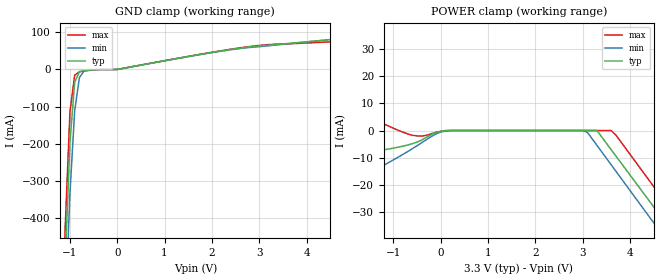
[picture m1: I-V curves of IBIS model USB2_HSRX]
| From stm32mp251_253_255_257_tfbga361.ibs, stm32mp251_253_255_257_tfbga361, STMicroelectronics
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[Model] USB2_HSRX
Model_type   Input
Polarity   Non-Inverting
Enable   Active-High
C_comp   5.492pF   5.368pF   5.494pF
Vinh = 150.000mV
Vinl = -150.000mV
[Model Spec]
[Receiver Thresholds]
Vcross_low = 0
Vcross_high = 500mv
Vdiff_ac = 150mv
Vdiff_dc = 100mv
Tdiffslew_ac = 1200ps
[Temperature Range]   25.000   125.000   -40.000
[Voltage Range]   3.300V   3.070V   3.630V
[GND Clamp Reference]   0.00V   0.00V   0.00V
[POWER Clamp Reference]   3.300V   3.070V   3.630V
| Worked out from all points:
|   GND clamp passes 1 mA (typ) near -0.53 V on its own axis
|   POWER clamp passes 1 mA (typ) near -0.14 V on its own axis
[GND Clamp]
-3.3V     -10.95A    -10.55A    -11.25A
-1.2V     -915.3mA   -1.032A    -838.8mA
-1.1V     -519.2mA   -657.5mA   -425.7mA
-1V       -197.7mA   -335.1mA   -115.1mA
-900mV    -35.05mA   -112.2mA   -15.67mA
-800mV    -5.949mA   -22.12mA   -6.454mA
-700mV    -2.647mA   -3.891mA   -4.243mA
-600mV    -1.536mA   -1.033mA   -2.639mA
1.971fV   0A         0A         0A
2V        45.55mA    45.52mA    46.3mA
3V        63.49mA    61.26mA    64.65mA
6.6V      104.1mA    107.2mA    86.72mA
[Power Clamp]
-3.3V     3.177A     2.138A     4.841A
-2.7V     505.5mA    62.8mA     1.908A
-2.6V     183.2mA    -5.843mA   1.435A
-2.4V     -6.294mA   -21.52mA   553.3mA
-2.2V     -8.53mA    -21.55mA   47.5mA
-2.1V     -8.617mA   -20.87mA   13.18mA
-2V       -8.548mA   -20.07mA   10.13mA
-900mV    -6.137mA   -9.8mA     96.78uA
3V        -8.976nA   -129.5nA   -7.302nA
3.6V      -7.035mA   -12.61mA   -9.228nA
4.7V      -32.83mA   -38.77mA   -25.41mA
6.6V      -77.39mA   -83.96mA   -70.53mA
